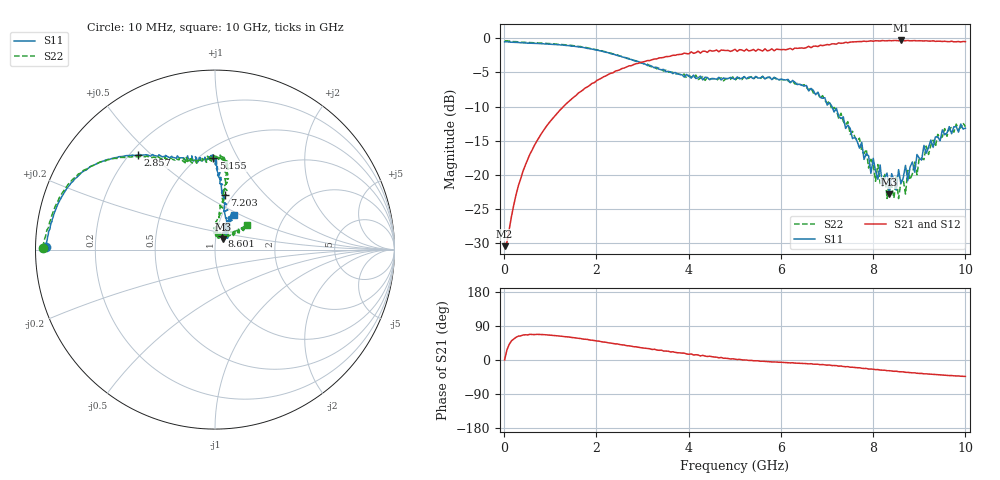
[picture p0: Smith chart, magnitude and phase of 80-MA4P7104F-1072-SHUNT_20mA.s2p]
!Agilent Technologies,E8364C,MY48140145,A.09.42.15
!Agilent E8364C: A.09.42.15
!Date: Wednesday, December 02, 2020 11:07:25
!Correction: S11(Full 2 Port(1,2))
!S21(Full 2 Port(1,2))
!S12(Full 2 Port(1,2))
!S22(Full 2 Port(1,2))
!S2P File: Measurements: S11, S21, S12, S22:
# Hz S  dB  R 50
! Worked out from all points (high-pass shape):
!   201 points, 10 MHz to 10 GHz, reference 50 ohm
!   highest |S21| = -0.31 dB at 8.601 GHz (marker M1); lowest = -30.4 dB at 10 MHz (marker M2)
!   |S21| within 3 dB of the highest: 3.083 GHz to end of sweep
!   lowest |S11| = -22.8 dB at 8.352 GHz (marker M3), VSWR 1.16, Z = 54.3 + j6.21 ohm
!   |S11| at or under -10 dB: 7.108 GHz to end of sweep
!   |S22| runs from -23.5 to -0.4 dB; largest |S21 - S12| = 0.031
!   S11 on the Smith chart (normalised r, x): 10 MHz: 0.03, +0.01; 2.857 GHz: 0.23, +0.45; 5.155 GHz: 0.58, +0.80; 7.203 GHz: 0.92, +0.61; 8.601 GHz: 1.07, +0.17; 10 GHz: 1.14, +0.46
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1e7  -0.52 179.2  -30.41 0.4  -33.05 -3.9  -0.39 179.3
2.5975e8  -0.61 174.6  -22.84 60.0  -22.87 59.9  -0.49 174.2
5.5945e8  -0.70 169.5  -16.94 67.9  -16.98 67.9  -0.62 169.0
1.7083e9  -1.33 150.0  -7.56 55.2  -7.51 55.6  -1.30 150.3
2.85715e9  -3.36 129.3  -3.72 34.9  -3.78 34.4  -3.28 130.7
3.35665e9  -4.51 119.6  -2.87 25.6  -2.96 26.2  -4.35 121.4
5.005e9  -5.99 91.5  -1.61 2.4  -1.54 1.7  -6.15 92.3
5.15485e9  -5.84 91.1  -1.70 0.5  -1.64 0.2  -6.03 89.8
6.7033e9  -7.63 88.0  -1.16 -11.0  -1.12 -10.2  -8.00 82.2
7.2028e9  -10.24 79.7  -0.85 -14.9  -0.82 -15.4  -10.47 82.5
7.95205e9  -19.76 58.8  -0.37 -23.8  -0.42 -24.4  -17.71 81.4
8.05195e9  -19.43 64.9  -0.35 -25.5  -0.37 -24.8  -20.92 81.9
8.25175e9  -20.38 42.1  -0.37 -26.9  -0.37 -27.5  -19.78 87.9
8.3017e9  -19.72 57.0  -0.36 -28.2  -0.29 -27.4  -23.43 83.5
8.35165e9  -22.81 51.9  -0.32 -28.2  -0.36 -28.8  -20.54 73.0
8.4016e9  -19.81 44.1  -0.36 -28.9  -0.32 -29.1  -21.67 88.7
8.55145e9  -19.22 50.9  -0.37 -30.8  -0.29 -30.5  -23.45 76.3
8.6014e9  -21.26 63.3  -0.31 -31.2  -0.37 -31.1  -21.06 56.1
8.7013e9  -18.60 58.7  -0.35 -32.5  -0.30 -31.7  -22.80 54.5
8.75125e9  -20.84 61.7  -0.32 -32.6  -0.35 -32.9  -19.32 53.2
9.1009e9  -15.67 62.2  -0.39 -36.5  -0.35 -35.6  -17.77 37.3
1e10  -13.15 61.4  -0.49 -43.3  -0.48 -43.5  -12.92 37.9
